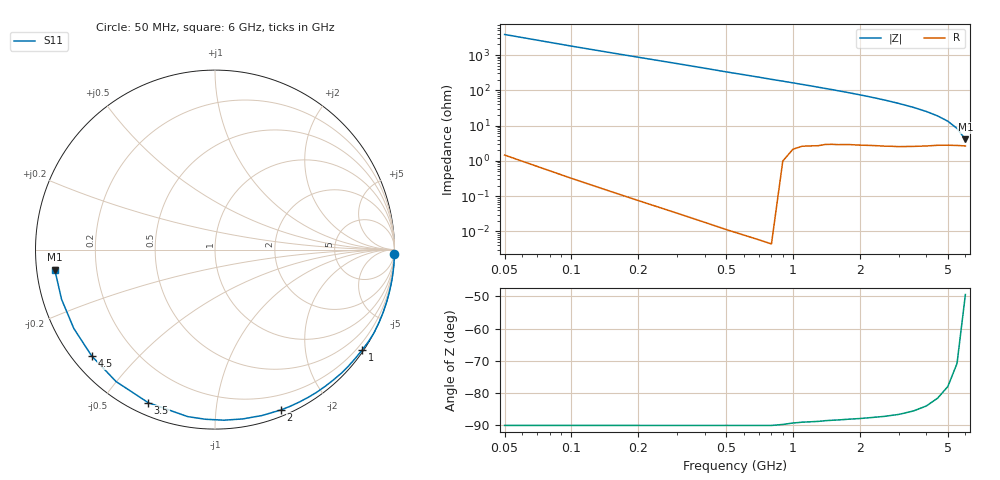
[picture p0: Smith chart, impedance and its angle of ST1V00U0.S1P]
! SIEMENS Discrete & RF Semiconductors
! BA892
! Si PIN Diode in SCD-80
! VR = 1 V
! S-Parameters:  September  1997
# GHz  S  MA  R  50
!  f  S11
! GHz  MAG  ANG
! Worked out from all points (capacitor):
!   34 points, 50 MHz to 6 GHz, reference 50 ohm
!   read as one part to ground: C = 889 fF near 50 MHz
!   lowest |Z| = 4.07 ohm at 6 GHz (marker M1)
!   S11 on the Smith chart (normalised r, x): 50 MHz: 0, -76; 1 GHz: 0.04, -3.25; 2 GHz: 0.06, -1.49; 3.5 GHz: 0.05, -0.65; 4.5 GHz: 0.06, -0.37; 6 GHz: 0.05, -0.06
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0.05  1 -1.5
0.15  1 -4.9
0.25  1 -8.3
0.4  1 -13.5
0.5  1 -17.1
0.6  1 -20.5
0.7  1 -23.9
0.8  1 -27.5
0.9  0.9972 -30.8
1  0.9926 -34.2
1.2  0.9871 -41.0
1.3  0.9848 -44.4
1.4  0.981 -47.8
1.5  0.9784 -51.0
1.6  0.9761 -54.5
1.8  0.9705 -61.1
2  0.9659 -67.7
2.2  0.9608 -74.2
2.4  0.9559 -80.7
2.6  0.9517 -87.0
2.8  0.9467 -93.3
3  0.9428 -99.3
3.5  0.9304 -113.6
4  0.9189 -126.9
4.5  0.9073 -139.2
5  0.9011 -150.8
5.5  0.8986 -162.1
6  0.8997 -172.9
